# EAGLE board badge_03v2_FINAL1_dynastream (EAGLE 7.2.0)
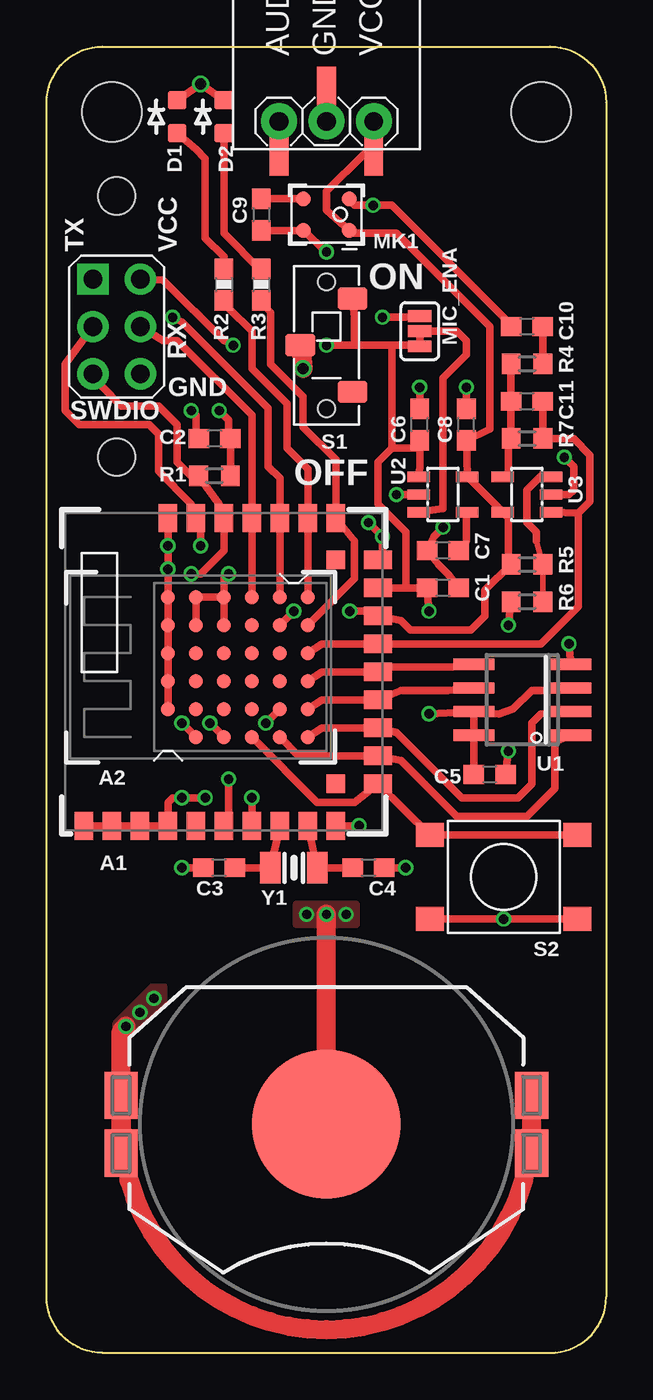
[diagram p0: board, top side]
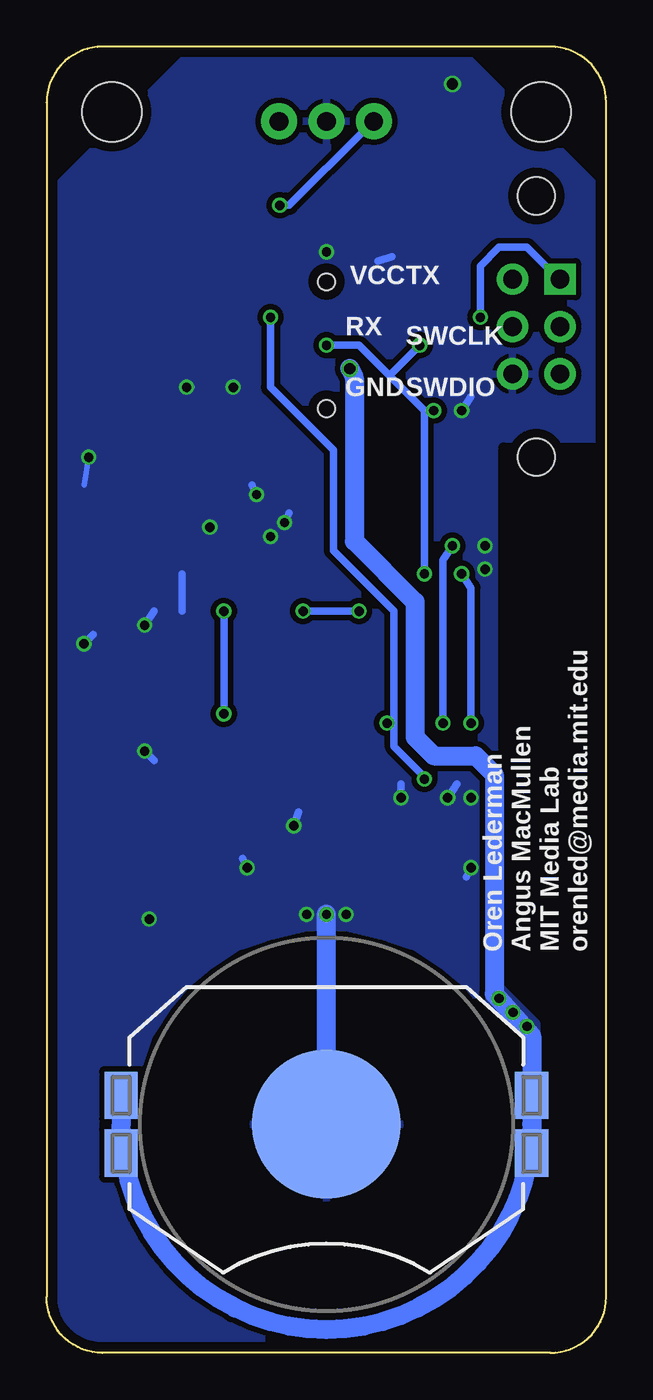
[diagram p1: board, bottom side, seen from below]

Size 30 x 70 mm. Coordinates in mm from the lower left corner, seen from the top.
Outline: 3,0 27,0 arc90 30,3 30,67 arc90 27,70 3,70 arc90 0,67 0,3 arc90 3,0
Copper layers (1*16): Top 0.035mm / dielectric 1.5mm / Bottom 0.035mm
Design rules "ITEADstudio_DRC *": minimum track width 6mil, minimum drill 12mil, track to track 6mil, track to pad 6mil, pad to pad 6mil, via to via 6mil, smd to smd 0mil, copper to edge 20mil, drill to drill 20mil, minimum pad ring 10mil, minimum via ring 6mil, stop-mask expansion 2mil, vias tented up to drill 100mil, thermal gap 10mil
Holes 2 mm at 3.75,48 3.75,62
Holes 3.2 mm at 3.5,66.5 26.5,66.5

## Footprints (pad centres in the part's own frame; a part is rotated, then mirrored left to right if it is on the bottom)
BMD-200 = smd 1.5 x 1: P$1 -8.25,7.5; P$2 -8.25,6; P$3 -8.25,4.5; P$4 -8.25,3; P$5 -8.25,1.5; P$6 -8.25,0; P$7 -8.25,-1.5; P$8 -8.25,-3; P$9 -8.25,-4.5; P$10 -8.25,-6; P$20 8.25,-6; P$21 8.25,-4.5; P$22 8.25,-3; P$23 8.25,-1.5; P$24 8.25,0; P$25 8.25,1.5; P$26 8.25,3 | smd 1 x 1.5: P$11 -6,-8.25; P$12 -4.5,-8.25; P$13 -3,-8.25; P$14 -1.5,-8.25; P$15 0,-8.25; P$16 1.5,-8.25; P$17 3,-8.25; P$18 4.5,-8.25; P$19 6,-8.25 | smd 1 x 1: P$27 -6,-6; P$28 6,-6
DYNASTREAM_N5 = smd 0.762 x 0.762: A2 1.5,0; A3 3,0; A4 4.5,0; A5 6,0; A6 7.5,0; B1 0,-1.5; B2 1.5,-1.5; B3 3,-1.5; B4 4.5,-1.5; B5 6,-1.5; B6 7.5,-1.5; C1 0,-3; C2 1.5,-3; C3 3,-3; C4 4.5,-3; C5 6,-3; C6 7.5,-3; D1 0,-4.5; D2 1.5,-4.5; D3 3,-4.5; D4 4.5,-4.5; D5 6,-4.5; D6 7.5,-4.5; E1 0,-6; E2 1.5,-6; E3 3,-6; E4 4.5,-6; E5 6,-6; E6 7.5,-6; F1 0,-7.5; F2 1.5,-7.5; F3 3,-7.5; F4 4.5,-7.5; F5 6,-7.5; F6 7.5,-7.5
ADMP401_SF_SMD = smd 1 x 2.51: AUD -2.54,-1.66; GND 0,1.66; VCC 2.54,-1.66 | drill 1 pad 1.93: AUDT -2.54,0; GNDT 0,0; VCCT 2.54,0
BATTCON_20MM_4LEGS_ISO = smd 1.778 x 2.54: 1 -11,1.55; 2 -11,-1.55; 3 11,1.55; 4 11,-1.55 | smd 8 x 8: NEG 0,0
BATTCON_20MM_4LEGS_ISO_NOCREAM = smd 1.778 x 2.54: 1 -11,1.55; 2 -11,-1.55; 3 11,1.55; 4 11,-1.55 | smd 8 x 8: NEG 0,0
C0603 = smd 1.1 x 1: 1 -0.85,0; 2 0.85,0
LED-0603 = smd 1 x 1: A 0,-0.877; C 0,0.877
TH_CONN_6 = drill 1 pad 1.676: GND 1.27,-2.54; RX 1.27,0; SWCLK -1.27,0; SWDIO -1.27,-2.54; VCC 1.27,2.54 | drill 1 pad 1.676 square: TX -1.27,2.54
PAD-JUMPER-3-2OF3_NC_BY_TRACE_YES_SILK_FULL_BOX = smd 0.635 x 1.27: 1 -0.813,0; 2 0,0; 3 0.813,0
MIC_SPU041X = smd 0.8 x 0.8: 1 0.85,1.23; 2 0.85,-1.23; 3 -0.85,-1.23; 4 -0.85,1.23
R0603 = smd 1 x 1.1: 1 -0.85,0; 2 0.85,0
0603-RES = smd 1.1 x 1: 1 -0.85,0; 2 0.85,0
CL-SB-12A-01 = smd 1.2 x 1.6: 1 -2.5,-1.4; 2 2.5,-1.4; C 0,1.4 | hole 0.9: -3.4,0; 3.4,0
TACT1 = smd 1.5 x 1.3: 1 -3.95,2.25; 2 3.95,2.25; 3 -3.95,-2.25; 4 3.95,-2.25
SOIC8 = smd 0.6 x 2.2: 1 -1.905,-2.6; 2 -0.635,-2.6; 3 0.635,-2.6; 4 1.905,-2.6; 5 1.905,2.6; 6 0.635,2.6; 7 -0.635,2.6; 8 -1.905,2.6
SOT23-5L = smd 0.55 x 1.2: 1 -0.95,-1.3; 2 0,-1.3; 3 0.95,-1.3; 4 0.95,1.3; 5 -0.95,1.3
CRYSTAL_2SMD = smd 1.1 x 1.7: P$1 -1.25,0; P$2 1.25,0

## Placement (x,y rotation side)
A1  BMD-200  [BMD-200]  9.5,36.5 90 top  (not fitted)
A2  DYNASTREAM_N5  [DYNASTREAM_N5]  6.5,33 90 top
A3  ADMP401_SF_GU  [ADMP401_SF_SMD]  15,66 0 top
BAT1  20mm coincell  [BATTCON_20MM_4LEGS_ISO]  15,12.25 0 top
BAT2  20mm coincell  [BATTCON_20MM_4LEGS_ISO_NOCREAM]  15,12.25 0 bottom
C1  10u  [C0603]  21.25,41 0 top  (not fitted)
C2  10u  [C0603]  9,49 180 top
C3  12p  [C0603]  9.25,26 180 top  (not fitted)
C4  12p  [C0603]  17.25,26 0 top  (not fitted)
C5  10u  [C0603]  23.75,31 0 top
C6  1u  [C0603]  20,49.75 90 top
C7  0.01u  [C0603]  21.25,43 180 top
C8  4.7u  [C0603]  22.5,49.75 90 top
C9  1u  [C0603]  11.5,61 270 top
C10  1u  [C0603]  25.75,55 0 top
C11  1n  [C0603]  25.75,51 0 top
D1  YL  [LED-0603]  7,66.25 0 top
D2  GR  [LED-0603]  9.5,66.25 0 top
J1  PROG_CONN_6  [TH_CONN_6]  3.75,55 0 top
MIC_ENA  DC/DC  [PAD-JUMPER-3-2OF3_NC_BY_TRACE_YES_SILK_FULL_BOX]  20,54.75 270 top
MK1  SPU0414(AMP)  [MIC_SPU041X]  15,61 270 top
R1  1k  [R0603]  9,47 180 top
R2  1k  [0603-RES]  9.5,57.25 270 top
R3  1k  [0603-RES]  11.5,57.25 270 top
R4  1k  [R0603]  25.75,53 0 top
R5  100k  [R0603]  25.75,42.25 180 top
R6  100k  [R0603]  25.75,40.25 0 top
R7  100k  [R0603]  25.75,49 180 top
S1  CL-SB-12A-01  [CL-SB-12A-01]  15,54 90 top
S2  TACT6MM4  [TACT1]  24.5,25.5 0 top
U1  AT25XE  [SOIC8]  25.5,35 90 top
U2  LP2985LV  [SOT23-5L]  21.25,46 270 top
U3  MCP6231  [SOT23-5L]  25.75,46 90 top
Y1  32768Hz  [CRYSTAL_2SMD]  13.25,26 180 top  (not fitted)

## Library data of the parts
A1 = rigado_BMD-200
A2 = dynastreamN5
A3 BAT1 BAT2 D1 D2 J1 MIC_ENA MK1 S1 S2 U1-U3 Y1 = Badge
C1-C11 R1 R4-R7 = rcl
R2 R3 = SparkFun-Passives

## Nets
BUTTON: A1.P$11 A2.D1 S2.1 S2.2
CS: A1.P$12 A2.E1 U1.1
GND: A1.P$1 A1.P$2 A1.P$3 A1.P$4 A1.P$7 A1.P$10 A1.P$19 A1.P$26 A2.A2 A2.A3 A2.A4 A2.A5 A2.A6 A3.GND A3.GNDT BAT1.NEG BAT2.NEG C1.2 C2.2 C3.2 C4.2 C5.2 C6.2 C7.2 C8.2 C9.2 D1.C D2.C J1.GND MK1.2 R6.1 S2.3 S2.4 U1.4 U2.2 U3.2
GRN: A1.P$20 A2.F5 R3.2
MIC_ENA: A1.P$6 A2.E2 MIC_ENA.1
MIC_F: A1.P$16 A2.F4 C11.2 R7.1 U3.1
MICVCC: A1.P$17 A2.E5 A3.VCC A3.VCCT C8.1 MK1.1 R5.2 U2.5 U3.5
MISO: A1.P$13 A2.F1 U1.2
MOSI: A1.P$15 A2.F3 U1.5
N$2: A1.P$8 C3.1 Y1.P$2
N$3: D1.A R2.1
N$4: D2.A R3.1
N$6: MIC_ENA.2 U2.3
N$7: C9.1 MK1.3
N$8: A1.P$9 C4.1 Y1.P$1
N$9: C7.1 U2.4
N$10: R5.1 R6.2 U3.3
N$11: A3.AUD A3.AUDT C10.1 MK1.4
N$13: C10.2 R4.2
N$14: C11.1 R4.1 R7.2 U3.4
RED: A1.P$21 A2.F6 R2.2
RX: A1.P$23 A2.D6 J1.RX
SCK: A1.P$14 A2.F2 U1.6
SWCLK: A1.P$25 A2.C1 J1.SWCLK
SWDIO: A1.P$24 A2.B1 J1.SWDIO R1.2
TX: A1.P$22 A2.E6 J1.TX
VBATT: BAT1.1 BAT1.2 BAT1.3 BAT1.4 BAT2.1 BAT2.2 BAT2.3 BAT2.4 S1.C
VCC: A1.P$18 A2.B5 A2.B6 A2.C5 A2.C6 C1.1 C2.1 C5.1 C6.1 J1.VCC MIC_ENA.3 R1.1 S1.2 U1.3 U1.7 U1.8 U2.1

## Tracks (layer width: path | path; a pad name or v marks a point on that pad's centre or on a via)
BUTTON
  Top 0.406: A2.D1 14.5,29.5 16.5,29.5 A1.P$11 S2.1 S2.2
CS
  Top 0.406: A2.E1 13.5,32 A1.P$12 19,31.75 22,28.75 25.75,28.75 27.25,30.25 27.25,32.75 U1.1
GND  (via drill 0.5, 0.6)
  Top 0.305: A3.GND A3.GNDT
  Top 0.406: U3.2 28,46 28.25,46.25 28.25,47.5 v27.75,48 | C3.2 v7.25,26 | A1.P$7 v11,29.75 | A1.P$10 v16.75,28.25 | C4.2 v19.25,26 | A1.P$1 A1.P$2 A1.P$3 A1.P$4 6.5,29.5 6.75,29.75 v7.25,29.75 v8.5,29.75 | R6.1 v24.75,39 | A1.P$19 18,43 v18,43.75 v17.25,44.5 | A1.P$26 v6.5,43.25 v6.5,42 A2.A6 A2.A5 A2.A4 A2.A3 A2.A2 | C6.2 v20,51.75 | C8.2 v22.5,51.75 | U2.2 v18.75,46 | D1.C v8.25,68 D2.C | v15,59 MK1.2 C9.2 | C5.2 v24.75,32.25 | U1.4 v28,38 | S2.4 v24.5,23.25 S2.3 | C2.2 8,49.5 8,50.25 v7.75,50.5 | v21.25,44.25 20.75,43.75 C7.2 21,42.25 21.5,41.75 C1.2
  Top 1.016: BAT2.NEG v15,23.5
  Bottom 0.305: v27.75,48 28,46.5
  Bottom 0.406: v7.25,26 7.5,25.5 | v11,29.75 11,30.5 | v16.75,28.25 16.5,29 | v19.25,26 19.5,26.5 | v24.75,39 24.25,39.75 | 22.75,41.75 22.75,39.75 | v17.25,44.5 17,45 | v8.5,29.75 8,30.5 | 11.5,58.75 12.25,58.5 | v20,51.75 20,52 | v22.5,51.75 22.25,51.75 | v18.75,46 19,46.5 | v24.75,32.25 24.25,31.75 | v28,38 27.5,38.5 | v7.75,50.5 7.25,51.25
  Bottom 1.016: BAT2.NEG v15,23.5
  other vias: 16.06,23.5 13.94,23.5
  pour Bottom (isolate 0.3, rank 2): 0,62 -0.5,0 30,0 30,62 22,70 8,70
  pour Top: 13.41,22.97 13.41,24.03 16.59,24.03 16.59,22.97
GRN
  Top 0.406: R3.2 12,55.75 12,53 13.75,51.25 13.75,49.62 15.5,47.88 A1.P$20 16.5,43.5 16.5,41.5 A2.F5
MIC_ENA  (via drill 0.5)
  Top 0.406: A1.P$6 9.75,29 v9.75,30.75 | MIC_ENA.1 19.25,55.5 v18,55.5 | A2.E2 v11.75,33.75
  Bottom 0.406: v9.75,30.75 9.88,31 11.38,32.5 11.38,33.25 11.38,33.75 | v18,55.5 18,51.75 14.62,48.38 14.62,43 11.38,39.75 11.38,33.75 | v11.75,33.75 11.38,33.75
MIC_F
  Top 0.305: 26.88,49 R7.1
  Top 0.406: C11.2 R7.1 | U3.1 28.5,45 | 28.5,45 29.12,45.62 29.12,48.12 28.25,49 26.88,49 | 28.5,45 28.5,40 26.5,38 A1.P$16 14.75,38 A2.F4
MICVCC  (via drill 0.5)
  Top 0.406: A3.VCCT A3.VCC 17,64.25 15,62.25 15,61.25 MK1.1 16.5,60 18.75,60 23.75,55 23.75,49.5 C8.1 U2.5 U3.5 24.75,44.75 24.75,42.75 R5.2 23.5,40.88 23.5,39.5 22.75,38.75 19.5,38.75 19,39.25 A1.P$17 17.5,39.75 v16.25,39.75 | A2.E5 v13.25,39.75
  Bottom 0.406: v13.25,39.75 v16.25,39.75
MISO
  Top 0.406: A2.F1 14.75,33.5 A1.P$13 18.75,33.25 22.25,29.75 25.25,29.75 26,30.5 26,33.75 26.5,34.25 U1.2
MOSI
  Top 0.406: A2.F3 14.75,36.5 A1.P$15 18.5,36.75 21.75,36.75 U1.5
N$2
  Top 0.406: A1.P$8 Y1.P$2 C3.1
N$3
  Top 0.406: R2.1 9.5,58.75 8.5,59.75 8.5,64 8,64.5 D1.A
N$4
  Top 0.406: D2.A 9.5,60 11.5,58 R3.1
N$6
  Top 0.406: U2.3 21.25,45.25 21.25,52.25 22.5,53.5 22.5,54.25 22,54.75 MIC_ENA.2
N$7
  Top 0.406: MK1.3 C9.1
N$8
  Top 0.406: A1.P$9 Y1.P$1 C4.1
N$9
  Top 0.406: U2.4 22.5,44.75 22.5,43.5 C7.1
N$10
  Top 0.305: R6.2 R5.1 26.25,43.5 | U3.3 26.5,47
  Top 0.406: 26.5,47 25.75,46.25 25.75,44.5 26.25,44 26.25,43.5
N$11  (via drill 0.5)
  Top 0.305: A3.AUD A3.AUDT
  Top 0.406: MK1.4 16.5,61.5 v17.5,61.5 18.5,61.5 24.75,55.25 C10.1
  Bottom 0.406: A3.AUDT 13,65.5 17,61.5 v17.5,61.5
N$13
  Top 0.406: C10.2 R4.2
N$14
  Top 0.305: R7.2 24.75,48.5 | 24.75,47.25 U3.4
  Top 0.406: R4.1 C11.1 R7.2 | 24.75,48.5 24.75,47.25
RED
  Top 0.406: R2.2 9.75,56 11,54.75 11,52.75 12.88,50.88 12.88,48.5 14,47.38 A1.P$21 A2.F6
RX
  Top 0.406: J1.RX 6.25,54.25 7,54.25 11,50.25 A1.P$23 A2.D6
SCK
  Top 0.406: A2.F2 14.75,35 A1.P$14 19,35.5 21.5,35.5 U1.6
SWCLK  (via drill 0.5)
  Top 0.406: J1.SWCLK 1,53 1,50.5 1.75,49.75 5.5,49.75 6,49.25 6,47.25 7.75,45.5 A1.P$25 8.25,44 v8.25,43.25 | v8.75,33.75 A2.C1
  Bottom 0.406: v8.25,43.25 8.75,42.5 v8.75,33.75
SWDIO  (via drill 0.5)
  Top 0.406: J1.SWDIO 3,51.75 4,50.75 6,50.75 7,49.75 7,47.75 7.75,47 R1.2 9.25,45.5 A1.P$24 9.5,43 8.25,41.75 v7.75,41.75 | A2.B1 v7.25,33.75
  Bottom 0.406: v7.25,33.75 7.25,41 v7.75,41.75
TX  (via drill 0.5)
  Top 0.406: v6.75,55.5 7.25,55.25 11.88,50.62 11.88,47.5 12.5,46.88 A1.P$22 A2.E6
  Bottom 0.406: v6.75,55.5 6.75,58.25 5.75,59.25 4.25,59.25 3,58 J1.TX
VBATT  (via drill 0.5, 0.6)
  Top 1.016: S1.C v13.75,52.75 | BAT2.3 4,12.25 arc90 15,1.25 arc90 26,12.25 | 26,12.25 BAT2.1 | BAT2.2 26,12.25 | BAT2.3 4,17.25 | 4,17.25 arc90 v4.25,17.5 4,17.25 | BAT2.4 BAT2.3
  Bottom 1.016: v13.75,52.75 13.5,52.25 13.5,43.5 10.25,40.25 10.25,33 9.25,32 7,32 6,31 6,19.25 4,17 BAT2.3 4,12.25 | 4,12.25 arc90 15,1.25 arc90 26,12.25 | BAT2.1 26,12.25 | BAT2.2 26,12.25 | 4,12.25 BAT2.4
  other vias: 5,18.25 5.75,19
  pour Bottom (isolate 0.254): 4,17 4,17.5 6,19.5 6,19
  pour Top: 4,17 4,17.5 6,19.5 6,19
VCC  (via drill 0.5)
  Top 0.406: A1.P$18 19.25,41 | 19.25,41 C1.1 v20.5,39.75 | 19.25,41 19.25,44 17.75,45.5 17.75,47.75 18.5,48.5 | U2.1 20,47.5 C6.1 19.75,48.5 18.5,48.5 | 18.5,54 18.5,48.5 | 18.5,54 19.25,54 MIC_ENA.3 | 16.5,54 18.5,54 | J1.VCC 6.25,57.5 9.5,54.25 v10,54 | U1.3 26.75,35.5 26,35.5 25,34.5 24.25,34.25 U1.7 | A2.B5 A2.B6 A2.C6 | A2.C5 A2.C6 | A2.C6 9.5,41.5 v9.75,41.75 | v20.5,34.25 U1.7 | U1.7 U1.8 C5.1 | v15,54 16.5,54 | 16.5,54 16.5,55.5 S1.2 | R1.1 C2.1 9.75,49.5 9.75,50 v9.25,50.5
  Bottom 0.406: 9.75,50.5 11.62,52.38 | 11.62,52.38 13.25,54 v15,54 | v10,54 11.62,52.38 | v9.75,41.75 9.75,50.5 | v9.25,50.5 9.75,50.5 | v20.5,34.25 v20.5,39.75

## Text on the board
tPlace: TX | VCC | ON | RX | GND | SWDIO | OFF
bPlace: TX | VCC | SWCLK | RX | SWDIO | GND | Oren Lederman / Angus MacMullen / MIT Media Lab / orenled@media.mit.edu

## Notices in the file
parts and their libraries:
SparkFun-Passives: Licensing: Creative Commons ShareAlike 4.0 International - https://creativecommons.org/licenses/by-sa/4.0
